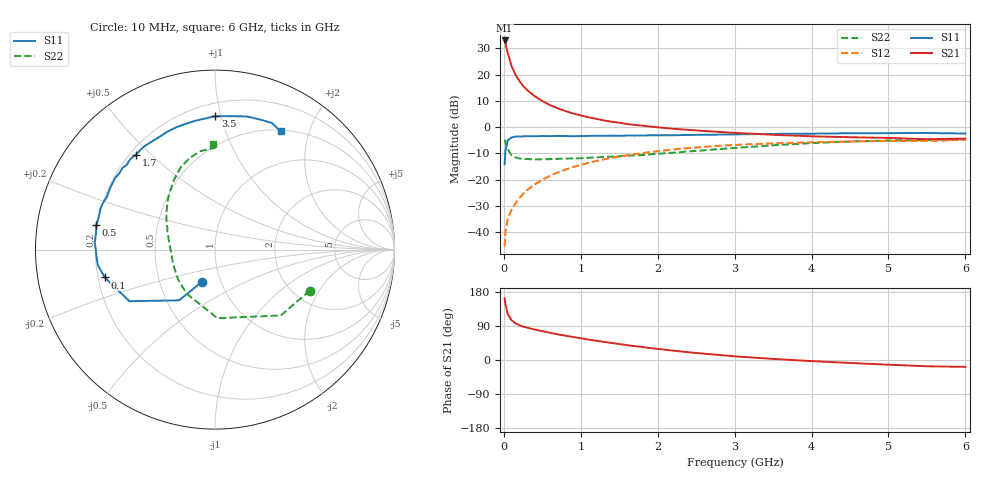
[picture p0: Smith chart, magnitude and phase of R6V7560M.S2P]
! SIEMENS Small Signal Semiconductors
! BFR193
! Si NPN RF Bipolar Junction Transistor in SOT23
! VCE = 0.75 V  IC = 60 mA
! Common Emitter S-Parameters:  May  1996
# GHz  S  MA  R  50
!  f  S11  S21  S12  S22
! GHz  MAG  ANG  MAG  ANG  MAG  ANG  MAG  ANG
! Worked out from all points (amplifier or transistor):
!   36 points, 10 MHz to 6 GHz, reference 50 ohm
!   highest |S21| = 33.0 dB at 10 MHz (marker M1)
!   |S21| within 3 dB of that: start of sweep to 36.12 MHz
!   unconditionally stable (mu >= 1): start of sweep to 15.84 MHz; 151.7 MHz to end of sweep
!   at 250 MHz: K = 1.09, MAG = 18.8 dB, |S12| = -25.5 dB
!   at 1.4 GHz: K = 1.08, MAG = 5.1 dB, |S12| = -11.7 dB
!   at 6 GHz: K = 1.02, MAG = -0.7 dB, |S12| = -4.9 dB
!   S11 on the Smith chart (normalised r, x): 10 MHz: 0.81, -0.30; 100 MHz: 0.23, -0.12; 500 MHz: 0.20, +0.10; 1.7 GHz: 0.22, +0.45; 3.5 GHz: 0.29, +0.96; 6 GHz: 0.52, +1.57
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0.01  0.1945 -112.3  44.66 162.8  0.0054 69.6  0.5754 -23.4
0.02  0.3463 -125.3  39.97 148.0  0.0099 65.3  0.5188 -45.0
0.05  0.5566 -148.9  25.83 121.9  0.0179 58.5  0.3825 -87.9
0.1  0.6336 -165.8  14.64 104.9  0.0266 61.9  0.2921 -122.8
0.15  0.6592 -172.6  10.04 96.9  0.035 65.2  0.2653 -140.5
0.2  0.6619 -177.3  7.637 91.9  0.044 68.1  0.2526 -150.1
0.25  0.6654 179.2  6.095 88.2  0.0531 69.7  0.2479 -157.3
0.3  0.672 176.6  5.106 85.4  0.0626 70.8  0.2459 -161.8
0.4  0.6694 171.6  3.889 80.5  0.0812 71.2  0.2439 -168.7
0.5  0.6763 168.4  3.136 76.2  0.0993 70.9  0.2436 -173.9
0.6  0.6724 164.1  2.625 71.8  0.118 69.8  0.2455 -177.4
0.7  0.678 160.6  2.282 67.7  0.1365 68.5  0.2485 179.5
0.9  0.6702 154.3  1.822 60.7  0.1735 65.4  0.2531 173.8
1.1  0.6795 147.8  1.538 53.9  0.2083 62.0  0.2607 169.7
1.4  0.6875 138.6  1.267 45.0  0.259 56.3  0.274 163.0
1.7  0.6879 129.9  1.102 36.5  0.3049 50.7  0.2897 156.3
2.2  0.6989 117.3  0.93 24.7  0.3745 41.2  0.3248 146.4
3  0.7258 99.0  0.776 9.7  0.4577 26.5  0.4 129.8
3.5  0.7432 89.9  0.714 2.9  0.49 18.2  0.4501 120.6
4.5  0.7628 76.4  0.641 -7.8  0.5321 4.6  0.5301 105.3
5.5  0.7734 65.9  0.588 -16.6  0.5455 -7.6  0.5662 90.2
6  0.7536 61.0  0.605 -18.1  0.5721 -11.3  0.588 91.1
